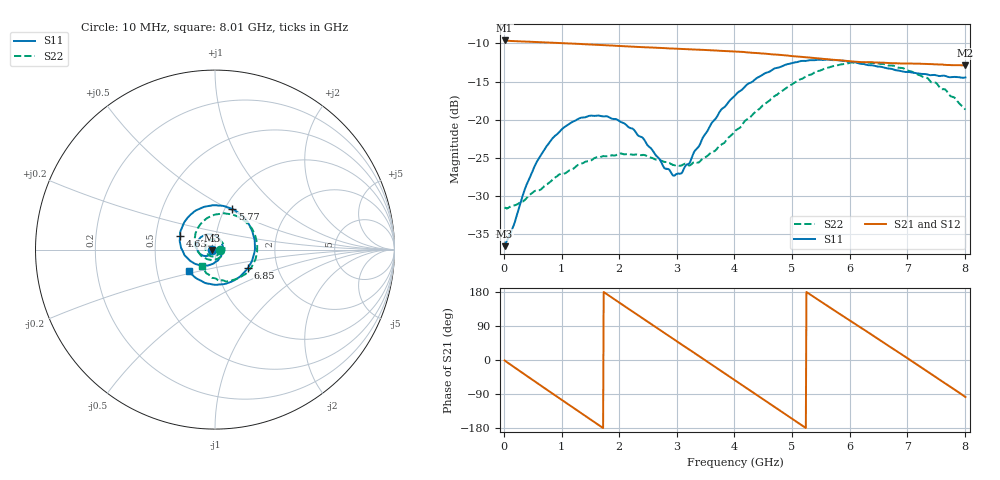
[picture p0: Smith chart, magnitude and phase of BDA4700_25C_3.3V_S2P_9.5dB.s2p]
!Agilent Technologies,E5071B,MY42404982,A.09.10
!Date: Mon Oct 20 18:06:59 2025
!Data & Calibration Information:
!Freq	S11:SOLT2(ON)	S21:SOLT2(ON)	S12:SOLT2(ON)	S22:SOLT2(ON)
# Hz S RI R 50
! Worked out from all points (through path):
!   801 points, 10 MHz to 8.01 GHz, reference 50 ohm
!   highest |S21| = -9.62 dB at 10 MHz (marker M1); lowest = -12.9 dB at 8.01 GHz (marker M2)
!   group delay of S21, straight-line fit = 283 ps
!   lowest |S11| = -36.6 dB at 10 MHz (marker M3), VSWR 1.03, Z = 48.5 - j0.136 ohm
!   |S11| at or under -10 dB: start of sweep to end of sweep
!   |S22| runs from -31.6 to -12.5 dB; largest |S21 - S12| = 0.0038
!   S11 on the Smith chart (normalised r, x): 10 MHz: 0.97, -0.00; 4.63 GHz: 0.67, +0.11; 5.77 GHz: 1.08, +0.52; 6.85 GHz: 1.41, -0.30; 8.01 GHz: 0.73, -0.18
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1e7  -0.0148 -0.00141  0.3304 -0.00727  0.3303 -0.00752  0.0267 -0.00136
4.1e8  -0.0272 -0.0279  0.2353 -0.2232  0.2352 -0.2235  0.0194 -0.0244
7.2e8  -0.0545 -0.0361  0.078 -0.3111  0.0782 -0.3111  -0.000855 -0.0373
1.02e9  -0.0848 -0.0227  -0.0933 -0.303  -0.0932 -0.3031  -0.0281 -0.0343
1.35e9  -0.1024 0.0134  -0.2443 -0.1954  -0.2444 -0.1956  -0.0511 -0.0065
1.93e9  -0.0619 0.08  -0.2843 0.1105  -0.2843 0.1105  -0.0256 0.0524
2.32e9  -0.00548 0.0792  -0.1446 0.2626  -0.1446 0.2627  0.0206 0.0554
2.68e9  0.036 0.0433  0.0408 0.2928  0.0403 0.2927  0.0499 0.0216
2.93e9  0.0432 0.00313  0.161 0.2444  0.1609 0.2438  0.0498 -0.00883
3.07e9  0.0393 -0.0209  0.2157 0.1954  0.2139 0.1968  0.0429 -0.0259
3.53e9  -0.02 -0.0818  0.2847 -0.0226  0.2849 -0.023  -0.00818 -0.0574
4.01e9  -0.1254 -0.0711  0.1655 -0.2257  0.166 -0.2251  -0.0768 -0.0341
4.32e9  -0.178 -0.0114  0.0219 -0.2734  0.0218 -0.2742  -0.1073 0.0146
4.63e9  -0.1942 0.0762  -0.1234 -0.2387  -0.1228 -0.2392  -0.1103 0.08
5e9  -0.1499 0.1808  -0.2366 -0.1103  -0.2372 -0.111  -0.0652 0.158
5.35e9  -0.0495 0.2405  -0.2499 0.0469  -0.2501 0.0455  0.0223 0.1978
5.77e9  0.0965 0.2261  -0.149 0.1958  -0.1486 0.1958  0.1457 0.1734
6.2e9  0.2008 0.1168  0.0215 0.2372  0.0246 0.2379  0.2275 0.0649
6.68e9  0.2104 -0.0499  0.1879 0.1411  0.1886 0.1409  0.2125 -0.0794
6.85e9  0.1831 -0.1029  0.2195 0.08  0.22 0.0786  0.1826 -0.1211
7.35e9  0.0431 -0.193  0.1999 -0.1171  0.2 -0.1174  0.0605 -0.1773
8.01e9  -0.1466 -0.1194  -0.0301 -0.2247  -0.0294 -0.225  -0.0736 -0.0904
